FUNCTION_BLOCK Example27_levitatelandspeed //2x1 flyways 1 xbot - LevitationLandw/Speed
VAR_INPUT
	Execute : BOOL;
END_VAR
VAR_OUTPUT
	Done : BOOL;
END_VAR
VAR_IN_OUT
	PM_Controller : PMControllerType;	// the planar motor controller to use
END_VAR
VAR
	levland_times : ARRAY[0..9] OF DINT;
	time_count : DINT;
	
	PMC_LevitationCtrlSpeed1 : PMC_LevitationCtrlSpeed;
	PMC_LevitationCtrlSpeed2 : PMC_LevitationCtrlSpeed;
	PMC_LevitationCtrlSpeed3 : PMC_LevitationCtrlSpeed;
	PMC_LevitationCtrlSpeed4 : PMC_LevitationCtrlSpeed;
	PMC_LevitationCtrlSpeed5 : PMC_LevitationCtrlSpeed;
	PMC_LevitationCtrlSpeed6 : PMC_LevitationCtrlSpeed;
	PMC_LevitationCtrlSpeed7 : PMC_LevitationCtrlSpeed;
	PMC_LevitationCtrlSpeed8 : PMC_LevitationCtrlSpeed;
	PMC_LevitationCtrlSpeed9 : PMC_LevitationCtrlSpeed;
	PMC_LevitationCtrlSpeed10 : PMC_LevitationCtrlSpeed;
END_VAR

//2x1 flyways 1 xbot - LevitationLandw/Speed

IF(Execute = TRUE)THEN
	time_count := time_count + 1;
ELSE
	time_count := 0;
END_IF;

//Land in 1.6s
PMC_LevitationCtrlSpeed1(Execute := Execute,XbotID := 1,Level := 0,Speed := 0,PM_Controller := PM_Controller);
IF(PMC_LevitationCtrlSpeed1.Done = TRUE AND PMC_LevitationCtrlSpeed2.Execute = FALSE)THEN
	levland_times[0] := time_count;
END_IF;

//Levitate in 1.6s
PMC_LevitationCtrlSpeed2(Execute := PMC_LevitationCtrlSpeed1.Done,XbotID := 1,Level := 1,Speed := 0,PM_Controller := PM_Controller);
IF(PMC_LevitationCtrlSpeed2.Done = TRUE AND PMC_LevitationCtrlSpeed3.Execute = FALSE)THEN
	levland_times[1] := time_count;
END_IF;

//Land in 0.8s
PMC_LevitationCtrlSpeed3(Execute := PMC_LevitationCtrlSpeed2.Done,XbotID := 1,Level := 0,Speed := 1,PM_Controller := PM_Controller);
IF(PMC_LevitationCtrlSpeed3.Done = TRUE AND PMC_LevitationCtrlSpeed4.Execute = FALSE)THEN
	levland_times[2] := time_count;
END_IF;

//Levitate in 0.8s
PMC_LevitationCtrlSpeed4(Execute := PMC_LevitationCtrlSpeed3.Done,XbotID := 1,Level := 1,Speed := 1,PM_Controller := PM_Controller);
IF(PMC_LevitationCtrlSpeed4.Done = TRUE AND PMC_LevitationCtrlSpeed5.Execute = FALSE)THEN
	levland_times[3] := time_count;
END_IF;

//Land in 0.4s
PMC_LevitationCtrlSpeed5(Execute := PMC_LevitationCtrlSpeed4.Done,XbotID := 1,Level := 0,Speed := 2,PM_Controller := PM_Controller);
IF(PMC_LevitationCtrlSpeed5.Done = TRUE AND PMC_LevitationCtrlSpeed6.Execute = FALSE)THEN
	levland_times[4] := time_count;
END_IF;

//Levitate in 0.4s
PMC_LevitationCtrlSpeed6(Execute := PMC_LevitationCtrlSpeed5.Done,XbotID := 1,Level := 1,Speed := 2,PM_Controller := PM_Controller);
IF(PMC_LevitationCtrlSpeed6.Done = TRUE AND PMC_LevitationCtrlSpeed7.Execute = FALSE)THEN
	levland_times[5] := time_count;
END_IF;

//Land in 0.2s
PMC_LevitationCtrlSpeed7(Execute := PMC_LevitationCtrlSpeed6.Done,XbotID := 1,Level := 0,Speed := 3,PM_Controller := PM_Controller);
IF(PMC_LevitationCtrlSpeed7.Done = TRUE AND PMC_LevitationCtrlSpeed8.Execute = FALSE)THEN
	levland_times[6] := time_count;
END_IF;

//Levitate in 0.2s
PMC_LevitationCtrlSpeed8(Execute := PMC_LevitationCtrlSpeed7.Done,XbotID := 1,Level := 1,Speed := 3,PM_Controller := PM_Controller);
IF(PMC_LevitationCtrlSpeed8.Done = TRUE AND PMC_LevitationCtrlSpeed9.Execute = FALSE)THEN
	levland_times[7] := time_count;
END_IF;

//Land in 0.1s
PMC_LevitationCtrlSpeed9(Execute := PMC_LevitationCtrlSpeed8.Done,XbotID := 1,Level := 0,Speed := 4,PM_Controller := PM_Controller);
IF(PMC_LevitationCtrlSpeed9.Done = TRUE AND PMC_LevitationCtrlSpeed10.Execute = FALSE)THEN
	levland_times[8] := time_count;
END_IF;

//Levitate in 0.1s
PMC_LevitationCtrlSpeed10(Execute := PMC_LevitationCtrlSpeed9.Done,XbotID := 1,Level := 1,Speed := 4,PM_Controller := PM_Controller);
IF(PMC_LevitationCtrlSpeed10.Done = TRUE AND Done = FALSE)THEN
	levland_times[9] := time_count;
END_IF;

Done := PMC_LevitationCtrlSpeed10.Done;

END_FUNCTION_BLOCK
